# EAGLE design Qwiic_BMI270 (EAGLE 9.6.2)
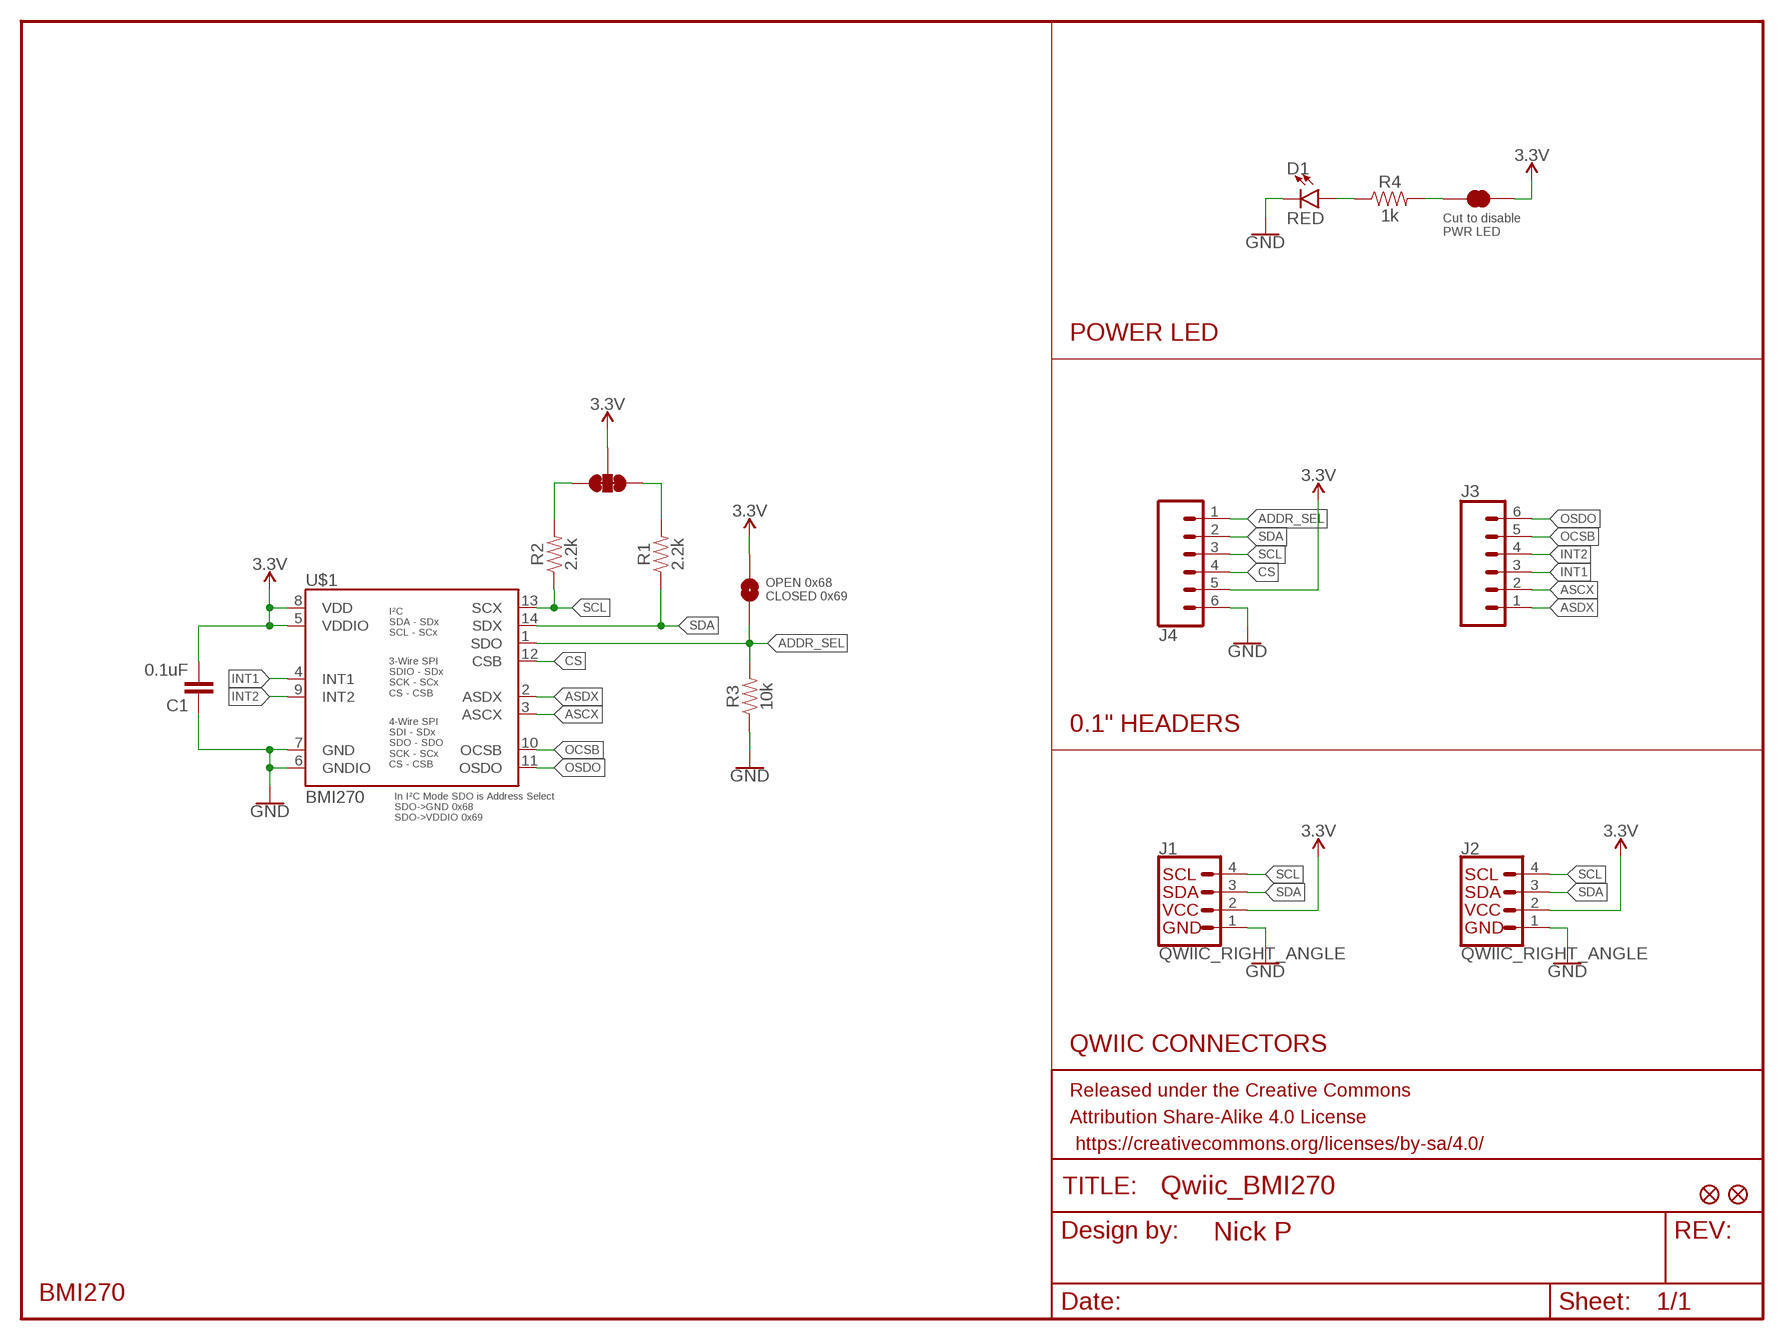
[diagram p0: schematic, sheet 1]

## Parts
C1  0.1uF  0.1UF-0603-25V-(+80/-20%)  [0603]
D1  RED  LED-RED0603  [LED-0603]
FD1  FIDUCIAL1X2  [FIDUCIAL-1X2]
FD2  FIDUCIAL1X2  [FIDUCIAL-1X2]
FRAME1  FRAME-LETTERNO_PACKAGE  [DUMMY]
J1  QWIIC_RIGHT_ANGLE  QWIIC_CONNECTORJS-1MM  [JST04_1MM_RA]
J2  QWIIC_RIGHT_ANGLE  QWIIC_CONNECTORJS-1MM  [JST04_1MM_RA]
J3  CONN_06NO_SILK_FEMALE_PTH  [1X06_NO_SILK]
J4  CONN_06NO_SILK_FEMALE_PTH  [1X06_NO_SILK]
JP1  JUMPER-SMT_3_2-NC_TRACE_SILK  [SMT-JUMPER_3_2-NC_TRACE_SILK]
JP2  JUMPER-SMT_2_NO_SILK  [SMT-JUMPER_2_NO_SILK]
JP3  JUMPER-SMT_2_NC_TRACE_SILK  [SMT-JUMPER_2_NC_TRACE_SILK]
R1  2.2k  2.2KOHM-0603-1/10W-1%  [0603]
R2  2.2k  2.2KOHM-0603-1/10W-1%  [0603]
R3  10k  10KOHM-0603-1/10W-1%  [0603]
R4  1k  1KOHM-0603-1/10W-1%  [0603]
U$1  BMI270  [BMI270]

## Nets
3.3V: C1.2 J1.2 J2.2 J4.5 JP1.2 JP2.2 JP3.2 U$1.5(VDDIO) U$1.8(VDD)
ADDR_SEL: J4.1 JP2.1 R3.2 U$1.1(SDO)
ASCX: J3.2 U$1.3(ASCX)
ASDX: J3.1 U$1.2(ASDX)
CS: J4.4 U$1.12(CSB)
GND: C1.1 D1.C J1.1 J2.1 J4.6 R3.1 U$1.6(GNDIO) U$1.7(GND)
INT1: J3.3 U$1.4(INT1)
INT2: J3.4 U$1.9(INT2)
N$1: JP1.1 R1.2
N$2: JP1.3 R2.2
N$3: JP3.1 R4.2
N$4: D1.A R4.1
OCSB: J3.5 U$1.10(OCSB)
OSDO: J3.6 U$1.11(OSDO)
SCL: J1.4 J2.4 J4.3 R2.1 U$1.13(SCX)
SDA: J1.3 J2.3 J4.2 R1.1 U$1.14(SDX)

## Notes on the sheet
- Cut to disable 
  PWR LED
- POWER LED
- OPEN 0x68
  CLOSED 0x69
- 0.1" HEADERS
- QWIIC CONNECTORS
- BMI270

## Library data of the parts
C1 = SparkFun-Capacitors:0.1UF: 0.1µF ceramic capacitors; PROD_ID: CAP-00810
D1 = SparkFun-LED:LED-RED: Red SMD LED; PROD_ID: DIO-00819
FD1 FD2 = SparkFun-Aesthetics:FIDUCIAL: Fiducial Alignment Points
FRAME1 = SparkFun-Aesthetics:FRAME-LETTER: Schematic Frame - Letter; DESIGNER: Nick P; VERSION: x01
J1 J2 = SparkFun-Connectors:QWIIC_CONNECTOR: SparkFun I2C Standard Qwiic Connector An SMD 1mm pitch JST connector makes it easy and quick (get it? Qwiic?) to connect I2C devices to each other. The Qwiic system enables fast and solderless connection between popular platforms and various sensors and actuators. We carry 200mm, 100mm, 50mm, and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; PROD_ID: CONN-13694
J3 J4 = SparkFun-Connectors:CONN_06: Multi connection point. Often used as Generic Header-pin footprint for 0.1 inch spaced/style header connections On any of the 0.1 inch spaced packages, you can populate with these: Break Away Headers - Straight (PRT-00116) Break Away Male Headers - Right Angle (PRT-00553) Female Headers (PRT-00115)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; PROD_ID: CONN-08437
JP1 = SparkFun-Jumpers:JUMPER-SMT_3_2-NC_TRACE: Normally closed trace jumper (2 of 2 connections) This jumper has a trace between all three pads so they are normally closed (NC). Use a razor knife to open the connection(s). For best results follow the IPC guidelines for cutting traces: Cutout at least 0.063 mm (0.005 in). Remove all loose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
JP2 = SparkFun-Jumpers:JUMPER-SMT_2_NO: Normally open jumper
JP3 = SparkFun-Jumpers:JUMPER-SMT_2_NC_TRACE: Normally closed trace jumper
R1 R2 = SparkFun-Resistors:2.2KOHM: 2.2kΩ resistor; PROD_ID: RES-08272
R3 = SparkFun-Resistors:10KOHM: 10kΩ resistor; PROD_ID: RES-00824
R4 = SparkFun-Resistors:1KOHM: 1kΩ resistor; PROD_ID: RES-07856
U$1 = SparkFun-Sensors:BMI270

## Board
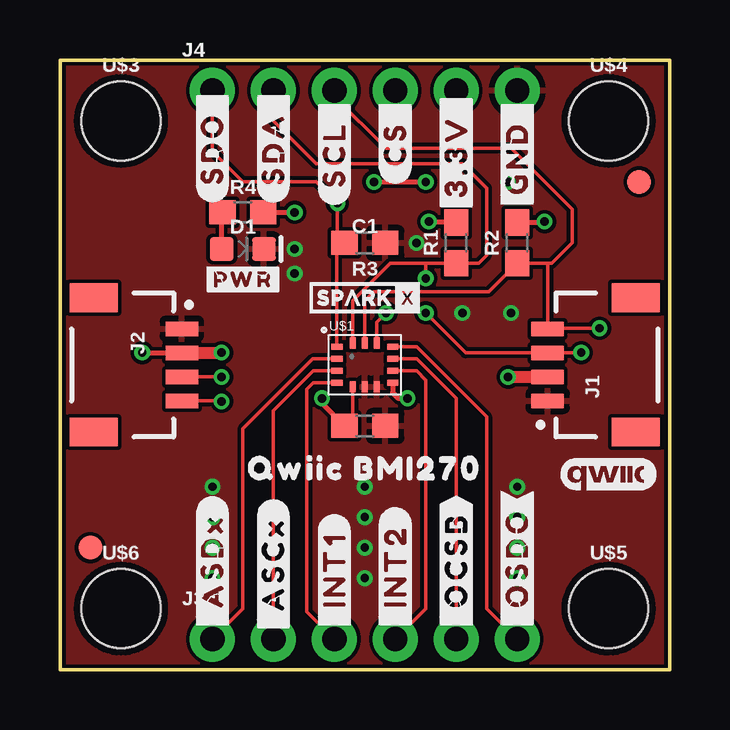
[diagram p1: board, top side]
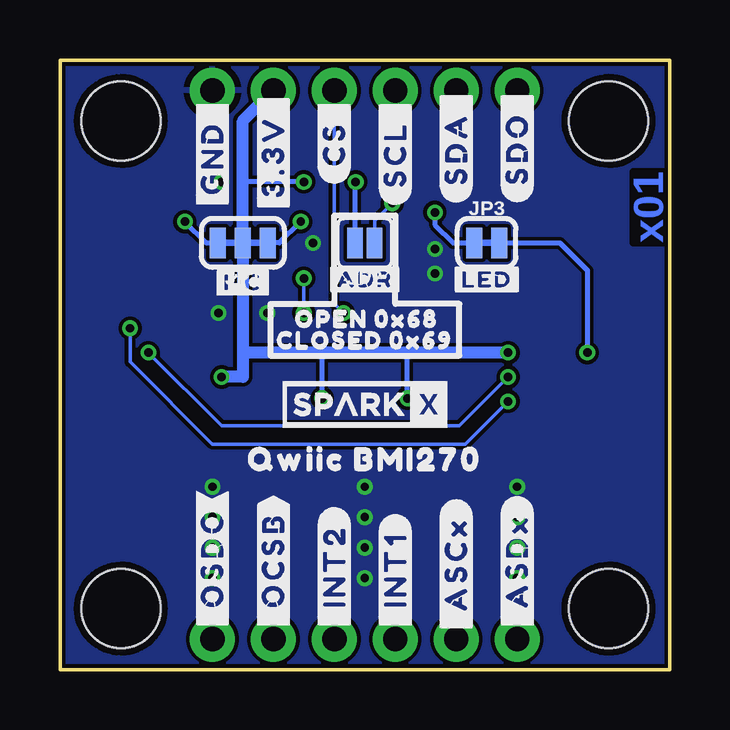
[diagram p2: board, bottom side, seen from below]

Size 25.4 x 25.4 mm. Coordinates in mm from the lower left corner, seen from the top.
Outline: 0,0 25.4,0 25.4,25.4 0,25.4 0,0
Copper layers (1*16): Top 0.035mm / dielectric 1.5mm / Bottom 0.035mm
Design rules "SparkFun-2-layer-PCBWay-LIMIT": minimum track width 6mil, minimum drill 0.3mm, track to track 6mil, track to pad 6mil, pad to pad 6mil, via to via 6mil, smd to smd 6mil, copper to edge 6mil, drill to drill 6mil, minimum pad ring 6mil, minimum via ring 6mil, stop-mask expansion 4mil, vias tented up to drill 25mil, thermal gap 10mil

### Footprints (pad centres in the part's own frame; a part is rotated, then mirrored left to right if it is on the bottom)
0603 = smd 1.1 x 1: 1 -0.85,0; 2 0.85,0
LED-0603 = smd 1 x 1: A -0.877,0; C 0.877,0
FIDUCIAL-1X2 = smd 1 x 1: 1 0,0
JST04_1MM_RA = smd 0.6 x 1.35: 1 -1.5,0; 2 -0.5,0; 3 0.5,0; 4 1.5,0 | smd 1.2 x 2: NC1 2.8,-3.675; NC2 -2.8,-3.675
1X06_NO_SILK = drill 1.016 pad 1.88: 1 0,0; 2 2.54,0; 3 5.08,0; 4 7.62,0; 5 10.16,0; 6 12.7,0
SMT-JUMPER_3_2-NC_TRACE_SILK = smd 0.66 x 1.27: 1 -1.041,0; 2 0,0; 3 1.041,0
SMT-JUMPER_2_NO_SILK = smd 0.635 x 1.27: 1 -0.406,0; 2 0.406,0
SMT-JUMPER_2_NC_TRACE_SILK = smd 0.66 x 1.27: 1 -0.521,0; 2 0.521,0
BMI270 = smd 0.475 x 0.25: 1 -1.163,0.748; 2 -1.163,0.247; 3 -1.163,-0.253; 4 -1.163,-0.752; 8 1.163,-0.75; 9 1.163,-0.25; 10 1.163,0.25; 11 1.163,0.75 | smd 0.25 x 0.475: 5 -0.497,-0.912; 6 0.003,-0.912; 7 0.502,-0.912; 12 0.502,0.91; 13 0.003,0.91; 14 -0.497,0.91
STAND-OFF = hole 3.302: 0,0

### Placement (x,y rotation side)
C1  12.7,10.16 180 top
D1  7.62,17.53 0 top
FD1  1.27,5.08 0 top
FD2  24.13,20.32 0 top
FRAME1  0,0 0 top
J1  20.32,12.7 90 top
J2  5.08,12.7 270 top
J3  6.35,1.27 0 top
J4  6.35,24.13 0 top
JP1  17.78,17.78 180 bottom
JP2  12.7,17.78 180 bottom
JP3  7.62,17.78 0 bottom
R1  16.51,17.78 90 top
R2  19.05,17.78 90 top
R3  12.7,17.78 180 top
R4  7.62,19.05 0 top
U$1  12.7,12.7 0 top
U$2  [#3#3V_#4]  16.51,24.13 90 top
U$3  [STAND-OFF]  2.54,22.86 0 top
U$4  [STAND-OFF]  22.86,22.86 0 top
U$5  [STAND-OFF]  22.86,2.54 0 top
U$6  [STAND-OFF]  2.54,2.54 0 top
U$7  [#GND_#4]  19.05,23.88 90 top
U$8  [#CS_#3]  13.97,23.88 90 top
U$9  [#SCL_#2]  11.43,23.88 90 top
U$10  [#SDA_#1]  8.89,24.26 90 top
U$11  [#SDO_#0]  6.35,24.26 90 top
U$12  [#_OSDO#8]  19.05,1.52 90 top
U$13  [#_OCSB#7]  16.51,1.52 90 top
U$14  [#_INT1#7]  11.43,1.52 90 top
U$15  [#_INT2#7]  13.97,1.52 90 top
U$16  [#_ASCX#5]  8.89,1.4 90 top
U$17  [#_ASDX#6]  6.35,1.52 90 top
U$18  [#PWR#2711]  7.62,16.26 0 top
U$19  [QWIIC_BMI2709]  12.7,8.38 0 top
U$20  [SPARKX-TINY]  12.7,15.49 0 top
U$21  [#I�C#2714]  17.78,16.13 0 bottom
U$22  [#LED#2712]  7.62,16.26 0 bottom
U$23  [#ADR#2713]  12.7,16.26 0 bottom
U$24  [OPEN_0X682714]  16.13,14.61 0 bottom
U$25  [CLOSED_0X692714]  16.89,13.72 0 bottom
U$26  [QWIIC_BMI2709]  12.7,8.76 0 bottom
U$27  [SPARKX-SMALL]  12.7,11.05 0 bottom
U$28  [#_OSDO#8]  19.05,1.52 90 bottom
U$29  [#_OCSB#7]  16.51,1.52 90 bottom
U$30  [#_INT2#7]  13.97,1.52 90 bottom
U$31  [#_INT1#7]  11.43,1.52 90 bottom
U$32  [#_ASCX#5]  8.89,1.4 90 bottom
U$33  [#_ASDX#6]  6.35,1.52 90 bottom
U$34  [#GND_#4]  19.05,23.88 90 bottom
U$35  [#3#3V_#4]  16.51,24.13 90 bottom
U$36  [#CS_#3]  13.97,23.88 90 bottom
U$37  [#SCL_#2]  11.43,23.88 90 bottom
U$38  [#SDA_#1]  8.89,24.26 90 bottom
U$39  [#SDO_#0]  6.35,24.26 90 bottom
U$41  [QWIIC_4MM]  22.86,8.13 0 top

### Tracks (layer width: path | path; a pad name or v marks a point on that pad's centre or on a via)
3.3V  (via drill 0.35)
  Top 0.152: U$1.5 12.2,10.16 C1.2 | J2.2
  Top 0.203: v3.43,13.21 J2.2 | C1.2 10.92,11.09 v10.92,11.3 | U$1.8 13.86,11.54 14.1,11.3 v14.48,11.3 | v13.08,20.32 v15.24,20.32
  Top 0.508: v18.67,12.19 v18.68,12.2 J1.2 | J2.2 v6.72,13.2 v6.73,13.21
  Bottom 0.203: JP3.2 4.57,17.78 3.43,16.64 v3.43,13.21 | v14.48,11.3 14.48,13.21 | v10.92,11.3 10.92,13.21 | JP2.2 13.11,20.3 v13.08,20.32 | v15.24,20.32 17.78,20.32
  Bottom 0.508: J4.5 17.78,22.86 17.78,20.32 JP1.2 17.78,13.21 | 17.78,13.21 17.78,12.19 v18.67,12.19 | v6.73,13.21 10.92,13.21 14.48,13.21 17.78,13.21
ADDR_SEL  (via drill 0.35)
  Top 0.152: U$1.1 11.54,17.78 R3.2 11.56,18.07 v11.56,19.43 10.67,20.32 7.62,20.32 6.35,21.59 J4.1
  Bottom 0.152: v11.56,19.43 12.29,18.69 JP2.1
ASCX
  Top 0.152: U$1.3 10.54,12.45 8.89,10.79 J3.2
ASDX
  Top 0.152: U$1.2 10.53,12.95 7.62,10.03 7.62,2.54 J3.1
CS  (via drill 0.35)
  Top 0.152: U$1.12 13.2,14.47 v13.59,14.86
  Bottom 0.152: v13.59,14.86 13.97,15.24 J4.4
GND  (via drill 0.35)
  other vias: 6.35,7.62 6.35,6.35 6.35,5.08 6.35,3.81 12.7,7.62 12.7,6.35 12.7,5.08 12.7,3.81 19.05,7.62 19.05,6.35 19.05,5.08 19.05,3.81 14.86,17.78 16.76,14.86 18.8,14.86 9.78,16.51 18.67,20.32 9.78,17.53
  pour Top: 0,0 25.4,0 25.4,25.4 0,25.4
  pour Bottom: 0,0 25.4,0 25.4,25.4 0,25.4
INT1
  Top 0.152: U$1.4 10.55,11.95 10.29,11.68 10.29,2.41 J3.3
INT2
  Top 0.152: J3.4 15.24,2.54 15.24,12.06 14.86,12.45 U$1.9
N$1  (via drill 0.35)
  Top 0.152: 15.41,18.63 v15.37,18.67
  Top 0.203: R1.2 15.41,18.63
  Bottom 0.203: v15.37,18.67 16.26,17.78 JP1.1
N$2  (via drill 0.35)
  Top 0.152: 20.15,18.63 v20.19,18.67
  Top 0.203: R2.2 20.15,18.63
  Bottom 0.203: v20.19,18.67 19.3,17.78 JP1.3
N$3  (via drill 0.35)
  Top 0.203: R4.2 v9.78,19.05
  Bottom 0.203: v9.78,19.05 9.78,18.54 9.02,17.78 JP3.1
N$4
  Top 0.203: D1.A 6.74,19.02 R4.1
OCSB
  Top 0.152: J3.5 16.51,11.3 14.86,12.95 U$1.10
OSDO
  Top 0.152: J3.6 17.78,2.54 17.78,10.54 14.86,13.46 13.87,13.46 U$1.11
SCL  (via drill 0.35)
  Top 0.152: U$1.13 12.7,15.37 13.08,15.75 17.87,15.75 R2.1 20.32,16.93 | 20.32,16.93 20.49,16.93 21.34,17.78 21.34,19.18 18.8,21.72 13.59,21.72 11.43,23.88 J4.3 | 20.32,16.93 J1.4 20.34,14.22 v22.48,14.22 | J2.4 6.71,11.2 v6.73,11.18
  Bottom 0.152: v6.73,11.18 8.51,9.4 19.05,9.4 22.48,12.83 v22.48,14.22
SDA  (via drill 0.35)
  Top 0.152: U$1.14 12.2,15.38 13.76,16.93 15.24,16.93 | 15.24,16.93 R1.1 17.44,16.93 17.78,17.27 17.78,20.07 16.76,21.08 10.67,21.08 8.89,22.86 J4.2 | v15.24,14.86 16.9,13.2 J1.3 21.71,13.2 v21.72,13.21 | v15.24,16.3 15.24,16.93 | J2.3 v6.72,12.2 v6.73,12.19
  Bottom 0.152: v15.24,14.86 v15.24,16.3 | v6.73,12.19 8.76,10.16 18.67,10.16 v21.72,13.21

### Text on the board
Bottom: x01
